ORGANIZATION_BLOCK OB 1
	VAR_TEMP
		TMPDUMMY	: INT;
		DTTEMP		: DATE_AND_TIME;
	END_VAR
BEGIN

	// Check forwarding of compound data type to FC
	// (This will create implicit DB pointers)
	AUF		DB 42
	LAR1		P##DTTEMP
	L		DW#16#12345678
	T		D [AR1, P#0.0]
	L		DW#16#87654321
	T		DBD 4
	L		DW#16#AABBCCDD
	T		D [AR1, P#4.0]
	L		DW#16#DDCCBBAA
	T		DBD 8
	CALL		FC 1 (
		DTTEMP	:= #DTTEMP,
		DTDB	:= DB42.DTVAR1,
	)

	// Check forwarding of compound data type from FB to FC
	CALL		FB 10, DB 10 (
		DUMMYIN	:= 42,
		DTVAR	:= DB42.DTVAR1,
	)


	// Check FB compound data type IN_OUT parameter semantics.
	L		42
	T		MW 0
	L		43
	T		MW 2
	L		44
	T		MW 4
	AUF		DB 42
	L		DW#16#11223344 // DB42.DTVAR4
	T		DBD 30
	L		DW#16#55667788 // DB42.DTVAR4
	T		DBD 34
	CALL		FB 20, DB 20 (
		DTIN		:= DB42.DTVAR2,
		INTIN		:= MW 0,
		DTOUT		:= DB42.DTVAR3,
		INTOUT		:= MW 2,
		DTINOUT		:= DB42.DTVAR4,
		INTINOUT	:= MW 4,
	)
	// Check modified DTINOUT (DB42.DTVAR4)
	AUF		DB 42
	L		DBD 30
	__ASSERT==	__ACCU 1,	DW#16#12131415
	L		DBD 34
	__ASSERT==	__ACCU 1,	DW#16#16171819


	CALL SFC 46 // STOP CPU
END_ORGANIZATION_BLOCK


FUNCTION_BLOCK FB 20
	VAR_INPUT
		DTIN		: DATE_AND_TIME;
		INTIN		: INT;
	END_VAR
	VAR_OUTPUT
		DTOUT		: DATE_AND_TIME;
		INTOUT		: INT;
	END_VAR
	VAR_IN_OUT
		DTINOUT		: DATE_AND_TIME;
		INTINOUT	: INT;
	END_VAR
	VAR
		DTSTAT		: DATE_AND_TIME;
		INTSTAT		: INT;
	END_VAR
	VAR_TEMP
		DBNR		: INT;
	END_VAR
BEGIN
	// Check all variable addresses
	L		P##DTIN
	__ASSERT==	__ACCU 1,	P#DIX 0.0
	L		P##INTIN
	__ASSERT==	__ACCU 1,	P#DIX 8.0
	L		P##DTOUT
	__ASSERT==	__ACCU 1,	P#DIX 10.0
	L		P##INTOUT
	__ASSERT==	__ACCU 1,	P#DIX 18.0
	L		P##DTINOUT	// 6 byte DB-ptr
	__ASSERT==	__ACCU 1,	P#DIX 20.0
	L		P##INTINOUT
	__ASSERT==	__ACCU 1,	P#DIX 26.0
	L		P##DTSTAT
	__ASSERT==	__ACCU 1,	P#DIX 28.0
	L		P##INTSTAT
	__ASSERT==	__ACCU 1,	P#DIX 36.0

	// Check DTINOUT data (via DB ptr)
	L		P##DTINOUT
	LAR1
	L		W [AR1, P#0.0]	// Get DB-nr from DB-ptr
	T		#DBNR
	__ASSERT==	__ACCU 1,	42
	AUF		DB [#DBNR]
	L		D [AR1, P#2.0]	// Get address from DB-ptr
	LAR1
	__ASSERT==	__ACCU 1,	P#DBX 30.0

	L		D [AR1, P#0.0]	// Get DTINOUT data
	__ASSERT==	__ACCU 1,	DW#16#11223344
	L		D [AR1, P#4.0]	// Get DTINOUT data
	__ASSERT==	__ACCU 1,	DW#16#55667788

	// Modify DTINOUT data (via DB ptr)
	L		DW#16#12131415
	T		D [AR1, P#0.0]	// Write DTINOUT data
	L		DW#16#16171819
	T		D [AR1, P#4.0]	// Write DTINOUT data
END_FUNCTION_BLOCK


DATA_BLOCK DB 20
	FB 20
BEGIN
END_DATA_BLOCK


FUNCTION FC 1 : VOID
	VAR_INPUT
		DTTEMP		: DATE_AND_TIME;
		DTDB		: DATE_AND_TIME;
	END_VAR
	VAR_TEMP
		DBNR		: INT;
	END_VAR
BEGIN
	// Load #DTTEMP into AR1
	L		P##DTTEMP
	LAR1
	UD		DW#16#FF000000
	__ASSERT==	__ACCU 1,	DW#16#87000000
	// Check the DB-pointer pointed to by #DTTEMP
	L		W [AR1, P#0.0]
	__ASSERT==	__ACCU 1,	0 // DB-nr
	T		#DBNR
	L		D [AR1, P#2.0]
	__ASSERT==	__ACCU 1,	DW#16#87000010
	LAR2
	AUF		DB [#DBNR]
	// Check the actual values
	L		D [AR2, P#0.0]
	__ASSERT==	__ACCU 1,	DW#16#12345678
	L		D [AR2, P#4.0]
	__ASSERT==	__ACCU 1,	DW#16#AABBCCDD


	// Load #DTDB into AR1
	L		P##DTDB
	LAR1
	UD		DW#16#FF000000
	__ASSERT==	__ACCU 1,	DW#16#87000000
	// Check the DB-pointer pointed to by #DTDB
	L		W [AR1, P#0.0]
	__ASSERT==	__ACCU 1,	42 // DB-nr
	T		#DBNR
	L		D [AR1, P#2.0]
	__ASSERT==	__ACCU 1,	DW#16#84000020
	LAR2
	AUF		DB [#DBNR]
	// Check the actual values
	L		D [AR2, P#0.0]
	__ASSERT==	__ACCU 1,	DW#16#87654321
	L		D [AR2, P#4.0]
	__ASSERT==	__ACCU 1,	DW#16#DDCCBBAA
END_FUNCTION


FUNCTION_BLOCK FB 10
	VAR_INPUT
		DUMMYIN		: INT;
		DTVAR		: DATE_AND_TIME;
	END_VAR
BEGIN
	CALL FC 11 (
		DTIN	:= #DTVAR,
	)
END_FUNCTION_BLOCK


FUNCTION FC 11 : VOID
	VAR_INPUT
		DTIN		: DATE_AND_TIME;
	END_VAR
	VAR_TEMP
		DBNR		: INT;
	END_VAR
BEGIN
	// Load #DTDB into AR1
	L		P##DTIN
	LAR1
	UD		DW#16#FF000000
	__ASSERT==	__ACCU 1,	DW#16#87000000
	// Check the DB-pointer pointed to by #DTIN
	L		W [AR1, P#0.0]
	__ASSERT==	__ACCU 1,	10 // DB-nr
	T		#DBNR
	L		D [AR1, P#2.0]
	__ASSERT==	__ACCU 1,	DW#16#84000010
	LAR2
	AUF		DB [#DBNR]
	// Check the actual values
	L		D [AR2, P#0.0]
	__ASSERT==	__ACCU 1,	DW#16#87654321
	L		D [AR2, P#4.0]
	__ASSERT==	__ACCU 1,	DW#16#DDCCBBAA
END_FUNCTION


DATA_BLOCK DB 10
	FB 10
BEGIN
END_DATA_BLOCK


DATA_BLOCK DB 42
	STRUCT
		DUMMY1		: INT;			// DBX 0.0
		DUMMY2		: INT;			// DBX 2.0
		DTVAR1		: DATE_AND_TIME;	// DBX 4.0
		DUMMY3		: INT;			// DBX 12.0
		DTVAR2		: DATE_AND_TIME;	// DBX 14.0
		DTVAR3		: DATE_AND_TIME;	// DBX 22.0
		DTVAR4		: DATE_AND_TIME;	// DBX 30.0
	END_STRUCT;
BEGIN
END_DATA_BLOCK
